| TEXAS INSTRUMENTS INCORPORATED
| Standard Linear and Logic Group
| IBIS Model of SN74AHC245
| OCTAL BUS TRANSCEIVERS WITH 3-STATE OUTPUTS
| This file contains package information for the following:
|  SOIC 20-pin (DW) package as [Component] AHC245_DW
|  PDIP 20-pin (N) package as [Component] AHC245_N
|  SSOP 20-pin (DB) package as [Component] AHC245_DB
|  TVSOP 20-pin (DGV) package as [Component] AHC245_DGV
|  TSSOP 20-pin (PW) package as [Component] AHC245_PW
| This device can be powered at the following Vccs:
|  5 volt Vcc
|  3.3 volt Vcc
|  2.5 volt Vcc
| This file provides unique models under the [Model Selector] for each Vcc.
| For operation at a specific Vcc, select the appropriate model after each
| [Model Selector] keyword.
[IBIS Ver]   3.2
[Comment char]  |_char
[File Name]   sn74ahc245.ibs
[File Rev]   1.0 | a_die
[Date]   July 12, 2001
[Source]   Data created from TI-SPICE simulations at TI-SLL.
[Notes]   The following is an IBIS list for the AHC245.
   Please contact sllibis@ti.com with questions and
   comments concerning SLL IBIS models.
   This IBIS model is created from a BA (back annotated netlist)
   -To comply with the data sheet we omitted the Vref
   and Rref from the Output Model
   -As there is no power clamp diode in the Input Model,
   we removed the Pwr Clamp table data from the Input Model
[Disclaimer] Property of Texas Instruments Incorporated.  Unauthorized
   reproduction and/or distribution is strictly prohibited.
   This product is protected under copyright law.
   Created  2001, (C) Copyright  2001, Texas Instruments
   Incorporated, All Rights Reserved
   UNLESS THERE IS A SIGNED, WRITTEN AGREEMENT TO THE
   CONTRARY, TEXAS INSTRUMENTS (TI) IS PROVIDING THE IBIS
   MODELS  AND WITHOUT ANY WARRANTY, EXPRESSED OR
   IMPLIED.  TI assumes no liability for:
   1) the accuracy of the IBIS models provided to your
   company;
   2) the proper functioning of these IBIS Models in your
   design or for any resulting applications; or
   3) infringement of patents, copyrights or intellectual
   property rights resulting from your use of these IBIS
   models.
   TI provides IBIS Models as a service to our customers.
   You and your company shall not distribute, sell or give
   these models to anyone else without prior written
   permission from TI.
   TI reserves the right to make changes to our products or
   to discontinue any semiconductor product or service
   without notice, and advises our customers to obtain the
   latest version of relevant information to verify, before
   placing orders, that the information being relied on is
   current.
   Please be aware that your receipt and use of the IBIS
   information provided shall serve as acceptance of these
   terms and conditions.  If you do not accept these terms,
   you should return or destroy the IBIS models and any
   other accompanying information immediately.
| Component AHC245_DW 20-pin SOIC
[Component]   AHC245_DW
[Manufacturer]   Texas Instruments, Inc.
[Package]
|   typ   min   max
R_pkg   3.800e-02   3.300e-02   4.500e-02
L_pkg   5.012e-09   4.110e-09   6.349e-09
C_pkg   7.170e-13   5.300e-13   8.680e-13
[Pin]   signal_name   model_name   R_pin   L_pin   C_pin
1   DIR   AHC245_DIR   4.200e-02   6.336e-09   8.650e-13
2   A1   AHC245_IO   4.300e-02   5.542e-09   8.670e-13
3   A2   AHC245_IO   3.400e-02   4.714e-09   7.320e-13
4   A3   AHC245_IO   3.400e-02   4.377e-09   5.910e-13
5   A4   AHC245_IO   3.600e-02   4.130e-09   5.330e-13
6   A5   AHC245_IO   3.500e-02   4.111e-09   5.300e-13
7   A6   AHC245_IO   3.400e-02   4.284e-09   5.830e-13
8   A7   AHC245_IO   3.400e-02   4.634e-09   7.260e-13
9   A8   AHC245_IO   4.000e-02   5.518e-09   8.650e-13
10   GND   GND   4.300e-02   6.349e-09   8.660e-13
11   B8   AHC245_IO   4.100e-02   6.281e-09   8.610e-13
12   B7   AHC245_IO   4.500e-02   5.561e-09   8.680e-13
13   B6   AHC245_IO   3.300e-02   4.778e-09   7.420e-13
14   B5   AHC245_IO   3.500e-02   4.414e-09   5.960e-13
15   B4   AHC245_IO   3.500e-02   4.110e-09   5.330e-13
16   B3   AHC245_IO   3.600e-02   4.130e-09   5.330e-13
17   B2   AHC245_IO   3.400e-02   4.377e-09   5.910e-13
18   B1   AHC245_IO   3.400e-02   4.714e-09   7.310e-13
19   NOE   AHC245_NOE   4.300e-02   5.569e-09   8.680e-13
20   VCC   POWER   4.200e-02   6.308e-09   8.640e-13
| Component AHC245_N 20-pin PDIP
[Component]   AHC245_N
[Manufacturer]   Texas Instruments, Inc.
[Package]
|   typ   min   max
R_pkg   4.300e-02   3.800e-02   5.000e-02
L_pkg   7.384e-09   4.680e-09   1.032e-08
C_pkg   5.100e-13   2.310e-13   8.210e-13
[Pin]   signal_name   model_name   R_pin   L_pin   C_pin
1   DIR   AHC245_DIR   4.200e-02   9.427e-09   8.100e-13
2   A1   AHC245_IO   4.600e-02   8.544e-09   4.560e-13
3   A2   AHC245_IO   4.800e-02   7.163e-09   4.350e-13
4   A3   AHC245_IO   4.000e-02   4.825e-09   2.610e-13
5   A4   AHC245_IO   4.000e-02   5.284e-09   6.480e-13
6   A5   AHC245_IO   4.000e-02   4.686e-09   2.320e-13
7   A6   AHC245_IO   4.000e-02   6.359e-09   4.890e-13
8   A7   AHC245_IO   3.800e-02   7.982e-09   4.750e-13
9   A8   AHC245_IO   4.300e-02   9.403e-09   4.750e-13
10   GND   GND   5.000e-02   1.032e-08   8.050e-13
11   B8   AHC245_IO   5.000e-02   1.028e-08   8.100e-13
12   B7   AHC245_IO   4.300e-02   9.383e-09   4.770e-13
13   B6   AHC245_IO   3.800e-02   7.978e-09   4.760e-13
14   B5   AHC245_IO   4.000e-02   6.302e-09   4.920e-13
15   B4   AHC245_IO   4.000e-02   4.680e-09   2.310e-13
16   B3   AHC245_IO   4.000e-02   5.284e-09   6.480e-13
17   B2   AHC245_IO   4.000e-02   4.822e-09   2.610e-13
18   B1   AHC245_IO   4.700e-02   7.118e-09   4.390e-13
19   NOE   AHC245_NOE   4.600e-02   8.492e-09   4.610e-13
20   VCC   POWER   4.300e-02   9.348e-09   8.210e-13
| Component AHC245_DB 20-pin SSOP
[Component]   AHC245_DB
[Manufacturer]   Texas Instruments, Inc.
[Package]
|   typ   min   max
R_pkg   4.000e-02   3.500e-02   5.100e-02
L_pkg   3.495e-09   3.035e-09   4.314e-09
C_pkg   4.200e-13   3.460e-13   5.020e-13
[Pin]   signal_name   model_name   R_pin   L_pin   C_pin
1   DIR   AHC245_DIR   4.900e-02   4.310e-09   5.020e-13
2   A1   AHC245_IO   4.800e-02   3.903e-09   4.870e-13
3   A2   AHC245_IO   3.500e-02   3.189e-09   3.960e-13
4   A3   AHC245_IO   3.500e-02   3.036e-09   3.470e-13
5   A4   AHC245_IO   3.500e-02   3.035e-09   3.670e-13
6   A5   AHC245_IO   3.500e-02   3.035e-09   3.670e-13
7   A6   AHC245_IO   3.500e-02   3.036e-09   3.470e-13
8   A7   AHC245_IO   3.500e-02   3.189e-09   3.970e-13
9   A8   AHC245_IO   4.700e-02   3.899e-09   4.880e-13
10   GND   GND   5.100e-02   4.314e-09   5.000e-13
11   B8   AHC245_IO   5.100e-02   4.314e-09   5.000e-13
12   B7   AHC245_IO   4.700e-02   3.899e-09   4.880e-13
13   B6   AHC245_IO   3.500e-02   3.189e-09   3.970e-13
14   B5   AHC245_IO   3.500e-02   3.036e-09   3.460e-13
15   B4   AHC245_IO   3.500e-02   3.035e-09   3.670e-13
16   B3   AHC245_IO   3.500e-02   3.035e-09   3.670e-13
17   B2   AHC245_IO   3.500e-02   3.036e-09   3.460e-13
18   B1   AHC245_IO   3.500e-02   3.189e-09   3.970e-13
19   NOE   AHC245_NOE   4.700e-02   3.899e-09   4.880e-13
20   VCC   POWER   5.100e-02   4.314e-09   5.020e-13
| Component AHC245_DGV 20-pin TVSOP
[Component]   AHC245_DGV
[Manufacturer]   Texas Instruments, Inc.
[Package]
|   typ   min   max
R_pkg   4.400e-02   3.800e-02   4.800e-02
L_pkg   2.561e-09   2.236e-09   2.961e-09
C_pkg   3.420e-13   2.640e-13   4.460e-13
[Pin]   signal_name   model_name   R_pin   L_pin   C_pin
1   DIR   AHC245_DIR   4.400e-02   2.935e-09   4.170e-13
2   A1   AHC245_IO   4.200e-02   2.869e-09   4.460e-13
3   A2   AHC245_IO   4.300e-02   2.399e-09   3.160e-13
4   A3   AHC245_IO   4.400e-02   2.236e-09   2.650e-13
5   A4   AHC245_IO   4.600e-02   2.278e-09   2.640e-13
6   A5   AHC245_IO   4.500e-02   2.274e-09   2.640e-13
7   A6   AHC245_IO   4.400e-02   2.285e-09   2.690e-13
8   A7   AHC245_IO   4.300e-02   2.452e-09   3.200e-13
9   A8   AHC245_IO   4.400e-02   2.900e-09   4.460e-13
10   GND   GND   4.400e-02   2.961e-09   4.180e-13
11   B8   AHC245_IO   4.500e-02   2.954e-09   4.180e-13
12   B7   AHC245_IO   4.200e-02   2.847e-09   4.430e-13
13   B6   AHC245_IO   4.500e-02   2.453e-09   3.190e-13
14   B5   AHC245_IO   4.500e-02   2.297e-09   2.690e-13
15   B4   AHC245_IO   4.800e-02   2.334e-09   2.680e-13
16   B3   AHC245_IO   4.800e-02   2.335e-09   2.670e-13
17   B2   AHC245_IO   4.600e-02   2.299e-09   2.680e-13
18   B1   AHC245_IO   4.600e-02   2.457e-09   3.200e-13
19   NOE   AHC245_NOE   4.300e-02   2.848e-09   4.410e-13
20   VCC   POWER   3.800e-02   2.812e-09   4.080e-13
| Component AHC245_PW 20-pin TSSOP
[Component]   AHC245_PW
[Manufacturer]   Texas Instruments, Inc.
[Package]
|   typ   min   max
R_pkg   4.500e-02   3.600e-02   5.700e-02
L_pkg   2.694e-09   2.290e-09   3.177e-09
C_pkg   1.560e-13   7.600e-14   2.590e-13
[Pin]   signal_name   model_name   R_pin   L_pin   C_pin
1   DIR   AHC245_DIR   3.600e-02   3.045e-09   2.590e-13
2   A1   AHC245_IO   5.100e-02   3.013e-09   1.890e-13
3   A2   AHC245_IO   4.400e-02   2.695e-09   1.640e-13
4   A3   AHC245_IO   4.700e-02   2.362e-09   7.900e-14
5   A4   AHC245_IO   4.700e-02   2.333e-09   8.600e-14
6   A5   AHC245_IO   4.700e-02   2.298e-09   8.500e-14
7   A6   AHC245_IO   4.700e-02   2.351e-09   7.900e-14
8   A7   AHC245_IO   4.400e-02   2.706e-09   1.650e-13
9   A8   AHC245_IO   4.900e-02   2.999e-09   1.880e-13
10   GND   GND   3.900e-02   3.039e-09   2.570e-13
11   B8   AHC245_IO   3.800e-02   3.044e-09   2.580e-13
12   B7   AHC245_IO   5.700e-02   3.177e-09   1.990e-13
13   B6   AHC245_IO   4.400e-02   2.825e-09   1.730e-13
14   B5   AHC245_IO   4.700e-02   2.429e-09   8.300e-14
15   B4   AHC245_IO   4.900e-02   2.383e-09   9.000e-14
16   B3   AHC245_IO   4.900e-02   2.347e-09   8.900e-14
17   B2   AHC245_IO   4.700e-02   2.290e-09   7.600e-14
18   B1   AHC245_IO   4.500e-02   2.613e-09   1.580e-13
19   NOE   AHC245_NOE   4.400e-02   2.883e-09   1.810e-13
20   VCC   POWER   3.900e-02   3.044e-09   2.560e-13
| Model AHC245_NOE
[Model Selector]   AHC245_NOE
AHC245_NOE_50   5 volt Vcc
AHC245_NOE_33   3.3 volt Vcc
AHC245_NOE_25   2.5 volt Vcc
| Model AHC245_DIR
[Model Selector]   AHC245_DIR
AHC245_DIR_50   5 volt Vcc
AHC245_DIR_33   3.3 volt Vcc
AHC245_DIR_25   2.5 volt Vcc
| Model AHC245_IO
[Model Selector]   AHC245_IO
AHC245_IO_50   5 volt Vcc
AHC245_IO_33   3.3 volt Vcc
AHC245_IO_25   2.5 volt Vcc
| Models and submodels in the file (9): AHC245_NOE_50 (Input), AHC245_NOE_33 (Input), AHC245_NOE_25 (Input), AHC245_DIR_50 (Input), AHC245_DIR_33 (Input), AHC245_DIR_25 (Input), AHC245_IO_50 (I/O), AHC245_IO_33 (I/O), AHC245_IO_25 (I/O)
